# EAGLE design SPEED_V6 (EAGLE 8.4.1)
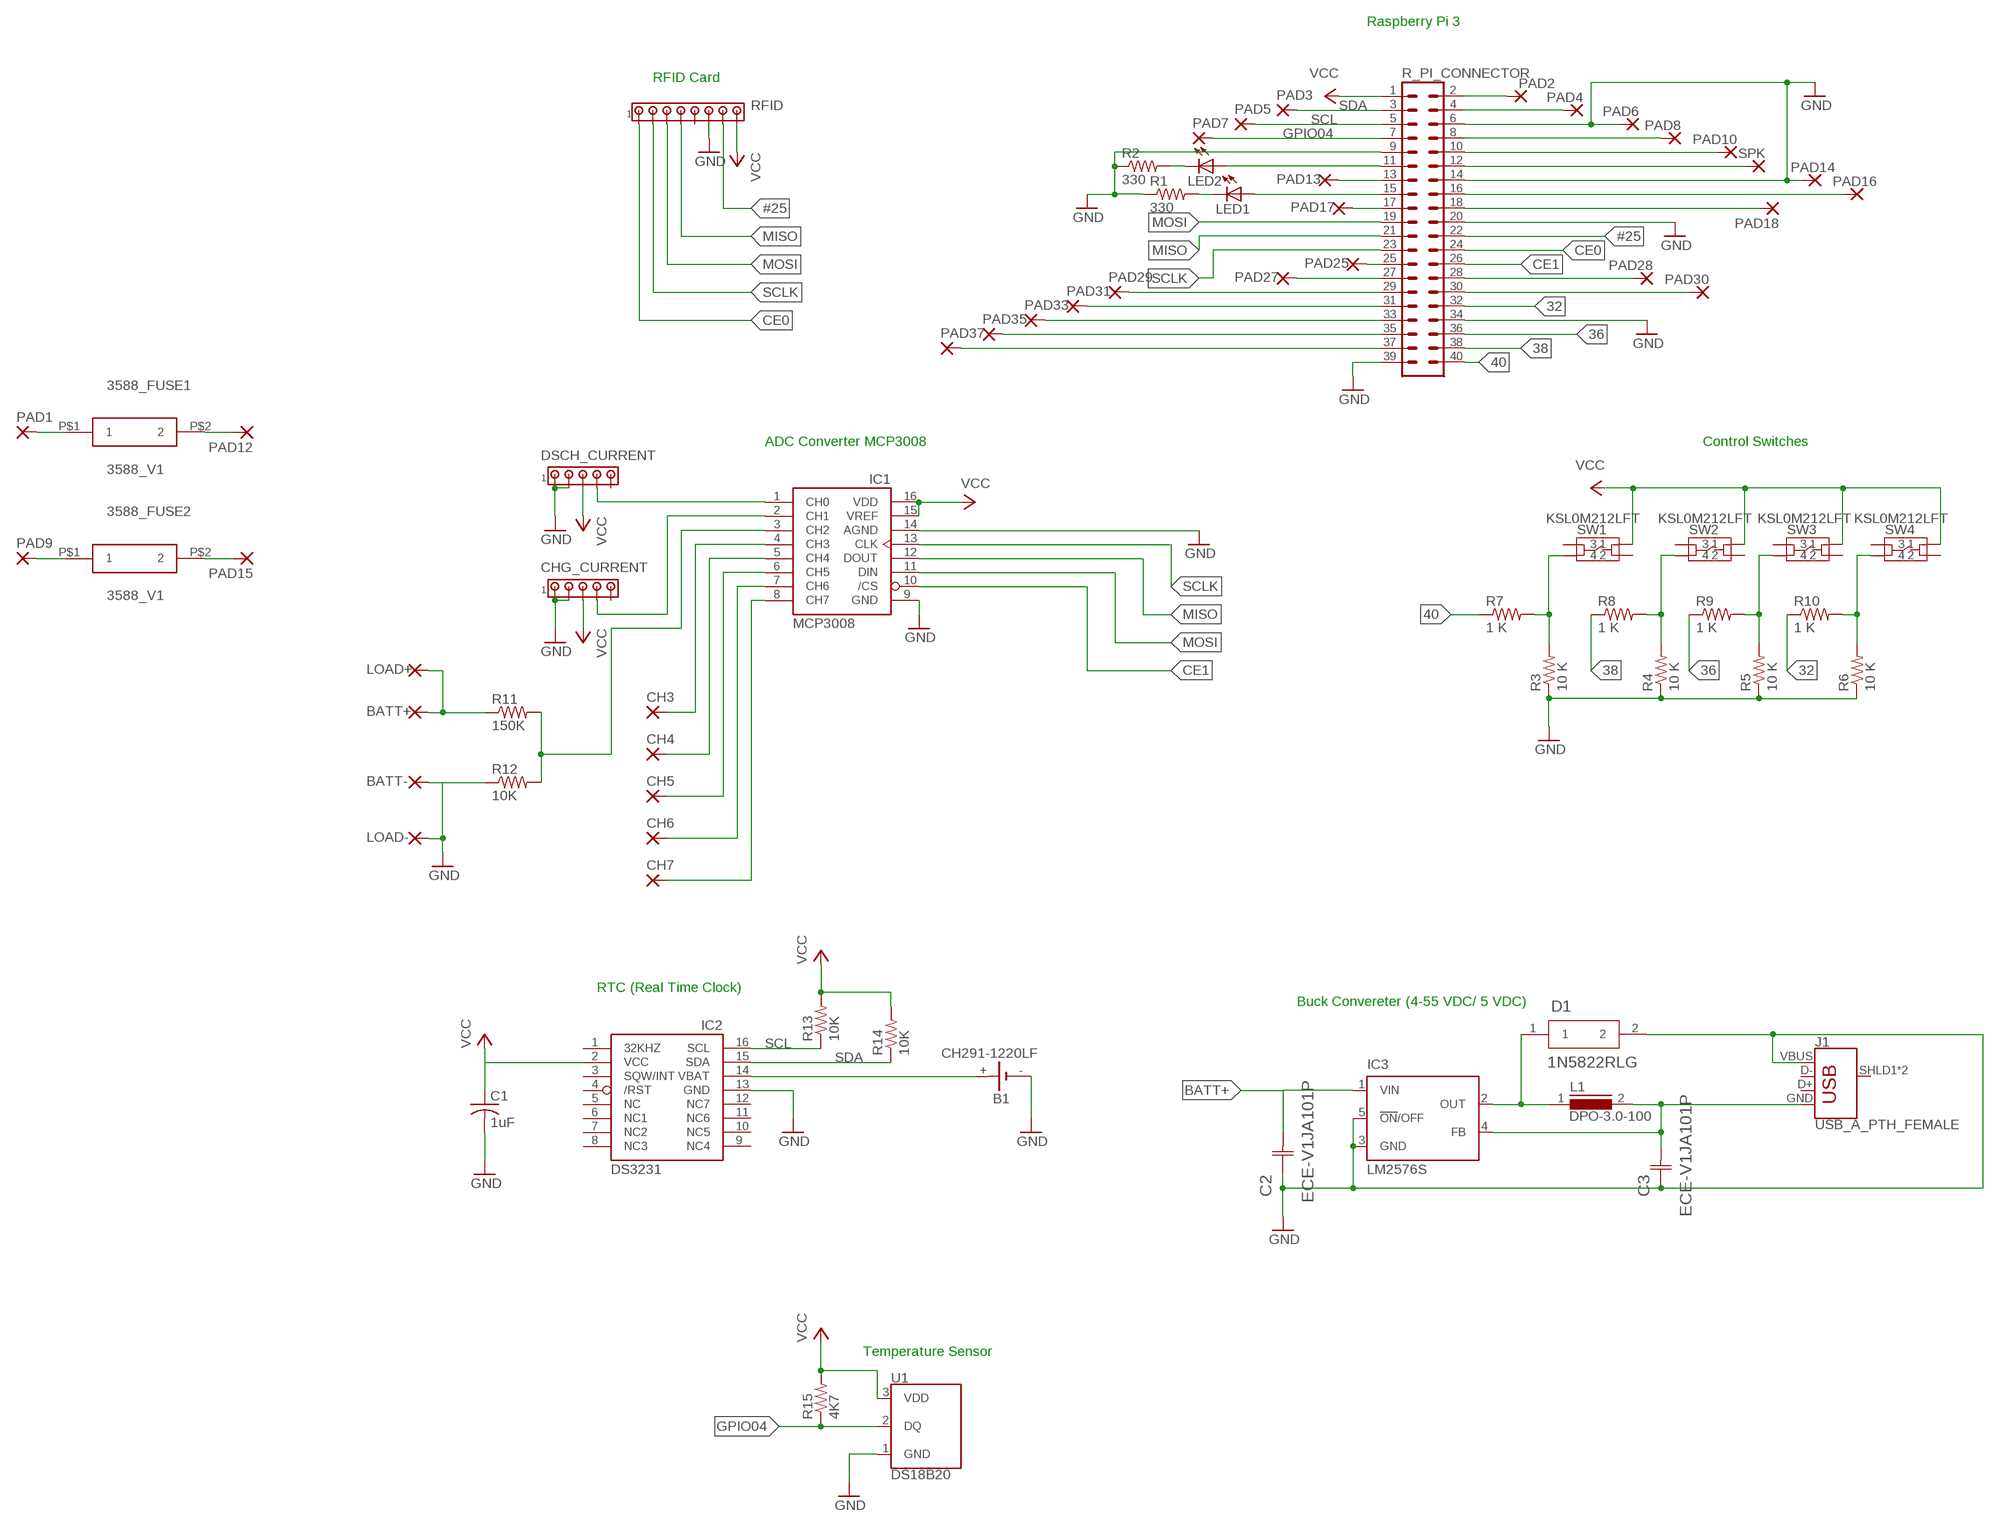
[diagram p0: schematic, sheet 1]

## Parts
3588_FUSE1  3588_V1  [3588_V1]
3588_FUSE2  3588_V1  [3588_V1]
B1  CH291-1220LF  [CH291-1220LF]
BATT+  3,81/1,4  [3,81/1,4]
BATT-  3,81/1,4  [3,81/1,4]
C1  1uF  C-USC0805  [C0805]
C2  ECE-V1JA101P  [CAP_ECEV_G]
C3  ECE-V1JA101P  [CAP_ECEV_G]
CH3  WIREPAD1,6/0,9  [1,6/0,9]
CH4  WIREPAD1,6/0,9  [1,6/0,9]
CH5  WIREPAD1,6/0,9  [1,6/0,9]
CH6  WIREPAD1,6/0,9  [1,6/0,9]
CH7  WIREPAD1,6/0,9  [1,6/0,9]
CHG_CURRENT  MTA05-100  [10X05MTA]
D1  1N5822RLG  [CASE_267-05]
DSCH_CURRENT  MTA05-100  [10X05MTA]
IC1  MCP3008  [DIL16]
IC2  DS3231/SO  [SO16W]
IC3  LM2576S  LM2596S  [TO263-5]
J1  USB_A_PTH_FEMALE  USB_A_PTH_MALE  [USB-A-H]
L1  DPO-3.0-100  ED26  [ED26]
LED1  LED5MM  [LED5MM]
LED2  LED5MM  [LED5MM]
LOAD+  3,81/1,4  [3,81/1,4]
LOAD-  3,81/1,4  [3,81/1,4]
PAD1  3,81/1,4  [3,81/1,4]
PAD2  1,6/0,9  [1,6/0,9]
PAD3  1,6/0,9  [1,6/0,9]
PAD4  1,6/0,9  [1,6/0,9]
PAD5  1,6/0,9  [1,6/0,9]
PAD6  1,6/0,9  [1,6/0,9]
PAD7  1,6/0,9  [1,6/0,9]
PAD8  1,6/0,9  [1,6/0,9]
PAD9  3,81/1,4  [3,81/1,4]
PAD10  1,6/0,9  [1,6/0,9]
PAD12  3,81/1,4  [3,81/1,4]
PAD13  1,6/0,9  [1,6/0,9]
PAD14  WIREPAD1,6/0,9  [1,6/0,9]
PAD15  3,81/1,4  [3,81/1,4]
PAD16  1,6/0,9  [1,6/0,9]
PAD17  1,6/0,9  [1,6/0,9]
PAD18  1,6/0,9  [1,6/0,9]
PAD25  1,6/0,9  [1,6/0,9]
PAD27  1,6/0,9  [1,6/0,9]
PAD28  1,6/0,9  [1,6/0,9]
PAD29  1,6/0,9  [1,6/0,9]
PAD30  1,6/0,9  [1,6/0,9]
PAD31  1,6/0,9  [1,6/0,9]
PAD33  1,6/0,9  [1,6/0,9]
PAD35  1,6/0,9  [1,6/0,9]
PAD37  1,6/0,9  [1,6/0,9]
R1  330  R-US_R1206  [R1206]
R2  330  R-US_R1206  [R1206]
R3  10 K  R-US_R1206  [R1206]
R4  10 K  R-US_R1206  [R1206]
R5  10 K  R-US_R1206  [R1206]
R6  10 K  R-US_R1206  [R1206]
R7  1 K  R-US_R1206  [R1206]
R8  1 K  R-US_R1206  [R1206]
R9  1 K  R-US_R1206  [R1206]
R10  1 K  R-US_R1206  [R1206]
R11  150K  R-US_R1206  [R1206]
R12  10K  R-US_R1206  [R1206]
R13  10K  R-US_R1206  [R1206]
R14  10K  R-US_R1206  [R1206]
R15  4K7  R-US_R1206  [R1206]
R_PI_CONNECTOR  SBH11-PBPC-D20  [SBH11-PBPC-D20]
RFID  MTA08-100  [10X08MTA]
SPK  WIREPAD1,6/0,9  [1,6/0,9]
SW1  KSL0M212LFT  [KSL0M212LFT_SWITCH]
SW2  KSL0M212LFT  [KSL0M212LFT_SWITCH]
SW3  KSL0M212LFT  [KSL0M212LFT_SWITCH]
SW4  KSL0M212LFT  [KSL0M212LFT_SWITCH]
U1  DS18B20  [TO-92-AMMO]

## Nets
32: R10.1 R_PI_CONNECTOR.32
36: R9.1 R_PI_CONNECTOR.36
38: R8.1 R_PI_CONNECTOR.38
40: R7.1 R_PI_CONNECTOR.40
#25: R_PI_CONNECTOR.22 RFID.7
BATT+: BATT+.1(P) C2.2 IC3.1(VIN) LOAD+.1(P) R11.1
CE0: R_PI_CONNECTOR.24 RFID.1
CE1: IC1.10(/CS) R_PI_CONNECTOR.26
GND: B1.- BATT-.1(P) C1.2 C2.1 C3.1 CHG_CURRENT.1 CHG_CURRENT.2 D1.2 DSCH_CURRENT.1 DSCH_CURRENT.2 IC1.9(GND) IC1.14(AGND) IC2.13(GND) IC3.3(GND) IC3.5(!ON!/OFF) J1.VBUS LOAD-.1(P) PAD6.1(P) PAD14.1(P) R1.1 R2.1 R3.1 R4.1 R5.1 R6.1 R12.1 R_PI_CONNECTOR.6 R_PI_CONNECTOR.9 R_PI_CONNECTOR.14 R_PI_CONNECTOR.20 R_PI_CONNECTOR.34 R_PI_CONNECTOR.39 RFID.6 U1.1(GND)
GPIO04: PAD7.1(P) R15.1 R_PI_CONNECTOR.7 U1.2(DQ)
MISO: IC1.12(DOUT) R_PI_CONNECTOR.21 RFID.4
MOSI: IC1.11(DIN) R_PI_CONNECTOR.19 RFID.3
N$1: R_PI_CONNECTOR.12 SPK.1(P)
N$2: PAD28.1(P) R_PI_CONNECTOR.28
N$3: LED1.K(C) R1.2
N$4: LED1.A R_PI_CONNECTOR.15
N$5: R6.2 R10.2 SW4.P$4
N$6: DSCH_CURRENT.4 IC1.1(CH0)
N$7: CHG_CURRENT.4 IC1.2(CH1)
N$8: IC1.3(CH2) R11.2 R12.2
N$9: PAD30.1(P) R_PI_CONNECTOR.30
N$10: PAD18.1(P) R_PI_CONNECTOR.18
N$11: PAD10.1(P) R_PI_CONNECTOR.10
N$12: PAD8.1(P) R_PI_CONNECTOR.8
N$13: 3588_FUSE1.P$1 PAD1.1(P)
N$14: D1.1 IC3.2(OUT) L1.1
N$15: PAD4.1(P) R_PI_CONNECTOR.4
N$16: R5.2 R9.2 SW3.P$4
N$17: LED2.A R_PI_CONNECTOR.11
N$18: LED2.K(C) R2.2
N$19: R4.2 R8.2 SW2.P$4
N$20: R3.2 R7.2 SW1.P$4
N$21: PAD2.1(P) R_PI_CONNECTOR.2
N$22: PAD13.1(P) R_PI_CONNECTOR.13
N$23: PAD17.1(P) R_PI_CONNECTOR.17
N$24: B1.+ IC2.14(VBAT)
N$25: PAD25.1(P) R_PI_CONNECTOR.25
N$26: PAD27.1(P) R_PI_CONNECTOR.27
N$27: PAD29.1(P) R_PI_CONNECTOR.29
N$28: PAD31.1(P) R_PI_CONNECTOR.31
N$29: PAD33.1(P) R_PI_CONNECTOR.33
N$30: PAD35.1(P) R_PI_CONNECTOR.35
N$31: PAD37.1(P) R_PI_CONNECTOR.37
N$32: PAD16.1(P) R_PI_CONNECTOR.16
N$33: 3588_FUSE1.P$2 PAD12.1(P)
N$34: CH3.1(P) IC1.4(CH3)
N$35: CH4.1(P) IC1.5(CH4)
N$36: CH5.1(P) IC1.6(CH5)
N$37: CH6.1(P) IC1.7(CH6)
N$38: CH7.1(P) IC1.8(CH7)
N$39: C3.2 IC3.4(FB) J1.GND L1.2
N$40: 3588_FUSE2.P$1 PAD9.1(P)
N$41: 3588_FUSE2.P$2 PAD15.1(P)
SCL: IC2.16(SCL) PAD5.1(P) R13.1 R_PI_CONNECTOR.5
SCLK: IC1.13(CLK) R_PI_CONNECTOR.23 RFID.2
SDA: IC2.15(SDA) PAD3.1(P) R14.1 R_PI_CONNECTOR.3
VCC: C1.1 CHG_CURRENT.3 DSCH_CURRENT.3 IC1.15(VREF) IC1.16(VDD) IC2.2(VCC) R13.2 R14.2 R15.2 R_PI_CONNECTOR.1 RFID.8 SW1.P$2 SW2.P$2 SW3.P$2 SW4.P$2 U1.3(VDD)
Unconnected: CHG_CURRENT.5 DSCH_CURRENT.5 IC2.1(32KHZ) IC2.3(SQW/INT) IC2.4(/RST) IC2.5(NC) IC2.6(NC1) IC2.7(NC2) IC2.8(NC3) IC2.9(NC4) IC2.10(NC5) IC2.11(NC6) IC2.12(NC7) J1.D+ J1.D- J1.SHLD1(SHIELD) J1.SHLD2(SHIELD) RFID.5 SW1.P$1 SW1.P$3 SW2.P$1 SW2.P$3 SW3.P$1 SW3.P$3 SW4.P$1 SW4.P$3

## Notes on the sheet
- Raspberry Pi 3
- RFID Card
- ADC Converter MCP3008 | Control Switches
- RTC (Real Time Clock)
- Buck Convereter (4-55 VDC/ 5 VDC)
- Temperature Sensor

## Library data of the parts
3588_FUSE1 3588_FUSE2 = costin_1:3588_V1
B1 = battery:CH291-1220LF: Battery Holder, SMT, 12mm
BATT+ = wirepad:3,81/1,4: THROUGH-HOLE PAD; SPICEPREFIX: X
BATT- LOAD+ LOAD- PAD1 PAD9 PAD12 PAD15 = wirepad:3,81/1,4: THROUGH-HOLE PAD
C1 = adafruit:C-US: CAPACITOR, American symbol
C2 C3 = digikey1:ECE-V1JA101P; MANUFACTURER_PART_NUMBER: ECEV1JA101P; VENDOR: Panasonic
CH3-CH7 PAD14 SPK = wirepad:WIREPAD: Wire PAD connect wire on PCB
CHG_CURRENT DSCH_CURRENT = con-amp:MTA05-100: AMP connector
D1 = digikey1:1N5822RLG; MANUFACTURER_PART_NUMBER: 1N5822RLG; VENDOR: ON Semiconductor
IC1 = adafruit:MCP3008
IC2 = adafruit:DS3231
IC3 = national-semiconductor:LM2596: SIMPLE SWITCHER® Power Converter 150 kHz 3A Step-Down Voltage Regulator Source: http://www.national.com/ds/LM/LM2596.pdf; MF: NATIONAL SEMICONDUCTOR; MPN: LM2596S-ADJ/NOPB; OC_FARNELL: 9494367; OC_NEWARK: 41K3842
J1 = SparkFun-Connectors:USB_A: USB-A Connector Male and female variants, as well as PTH and SMT variants SparkFun Products: SparkFun XBee Explorer Dongle PTH Male SparkFun MicroView-USB Programmer SMT Male SparkFun USB Type A Female Breakout SMT Female; PROD_ID: CONN-08367; SF_ID: PRT-00437; SPICEPREFIX: X
L1 = inductors:ED26: INDUCTOR; SPICEPREFIX: L
LED1 LED2 = adafruit:LED: LED
PAD2-PAD8 PAD10 PAD13 PAD16-PAD18 PAD25 PAD27-PAD31 PAD33 PAD35 PAD37 = wirepad:1,6/0,9: THROUGH-HOLE PAD
R1 R2 R11-R15 = adafruit:R-US_: RESISTOR, American symbol
R3-R6 = adafruit:R-US_: RESISTOR, American symbol; MPN: RC1206JR-0710KL; OC_NEWARK: 68R0303
R7-R10 = adafruit:R-US_: RESISTOR, American symbol; OC_NEWARK: unknown
R_PI_CONNECTOR = con-sullins:SBH11-PBPC-D20: HEADER - Vertical, Shrouded
RFID = con-amp:MTA08-100: AMP connector
SW1-SW4 = costin_1:KSL0M212LFT
U1 = SparkFun-Sensors:DS18B20: Dallas/Maxim DS18B20 1-Wire Temperature Sensor The DS18B20 reports degrees C with 9 to 12-bit precision, -55C to 125C (+/-0.5C). Each sensor has a unique 64-Bit Serial number etched into it - allows for a huge number of sensors to be used on one data bus. Datasheet SparkFun Products One Wire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; STORE_ID: SEN-00245

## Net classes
0 default: width 0.305 mm, drill 0.508 mm, clearance 0.254 mm

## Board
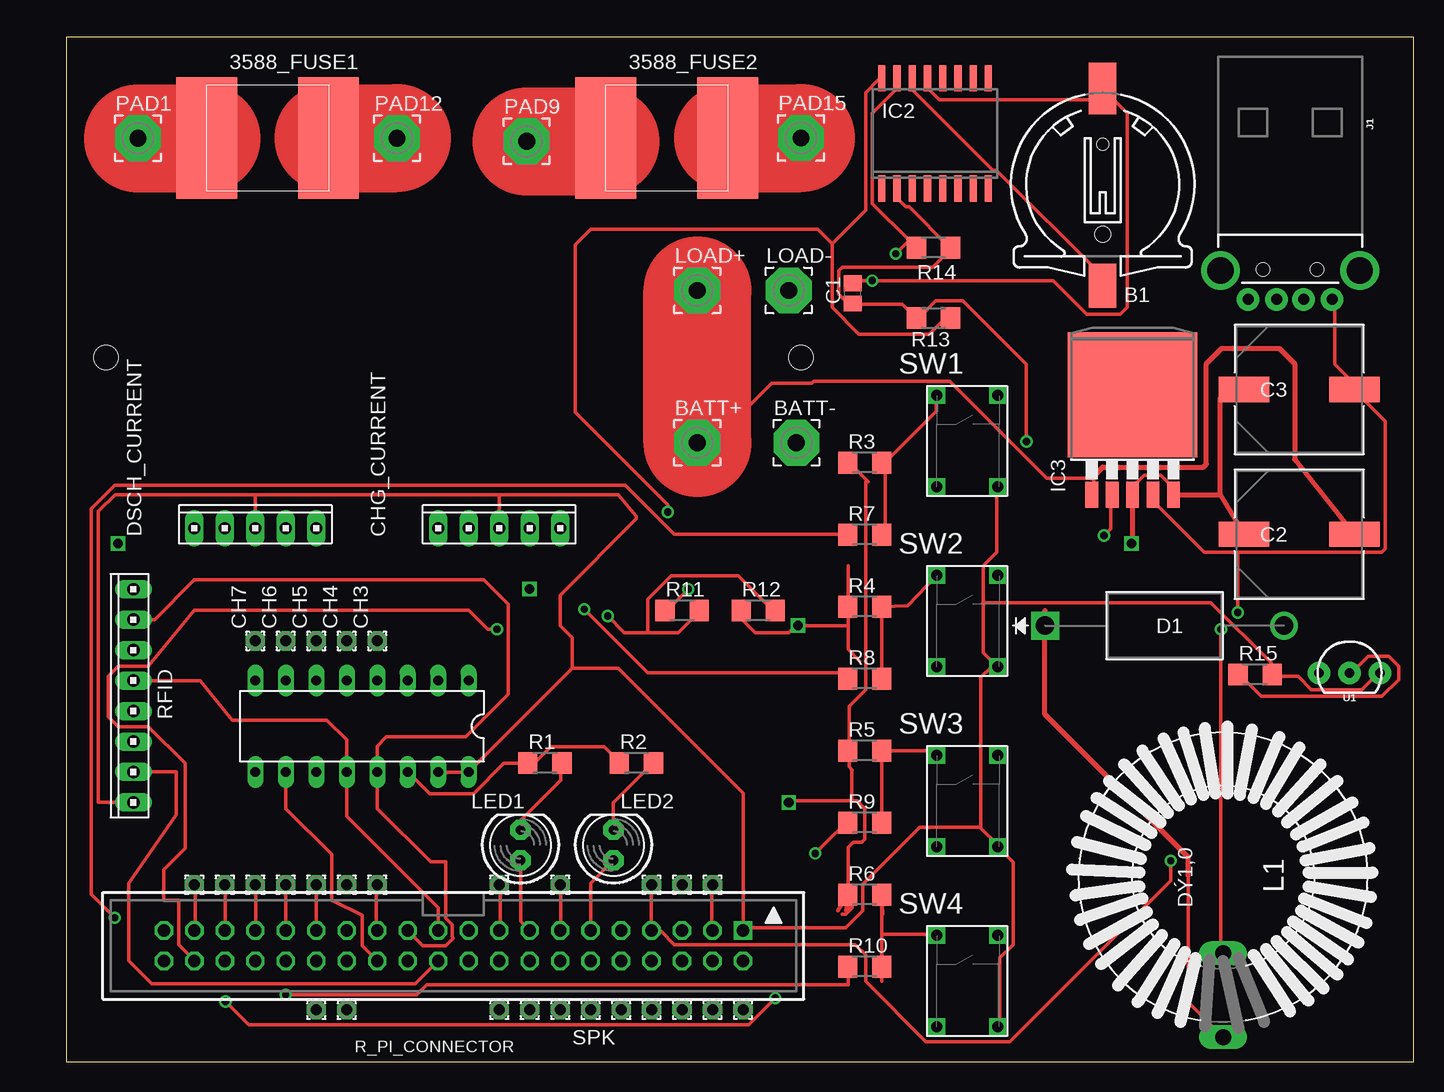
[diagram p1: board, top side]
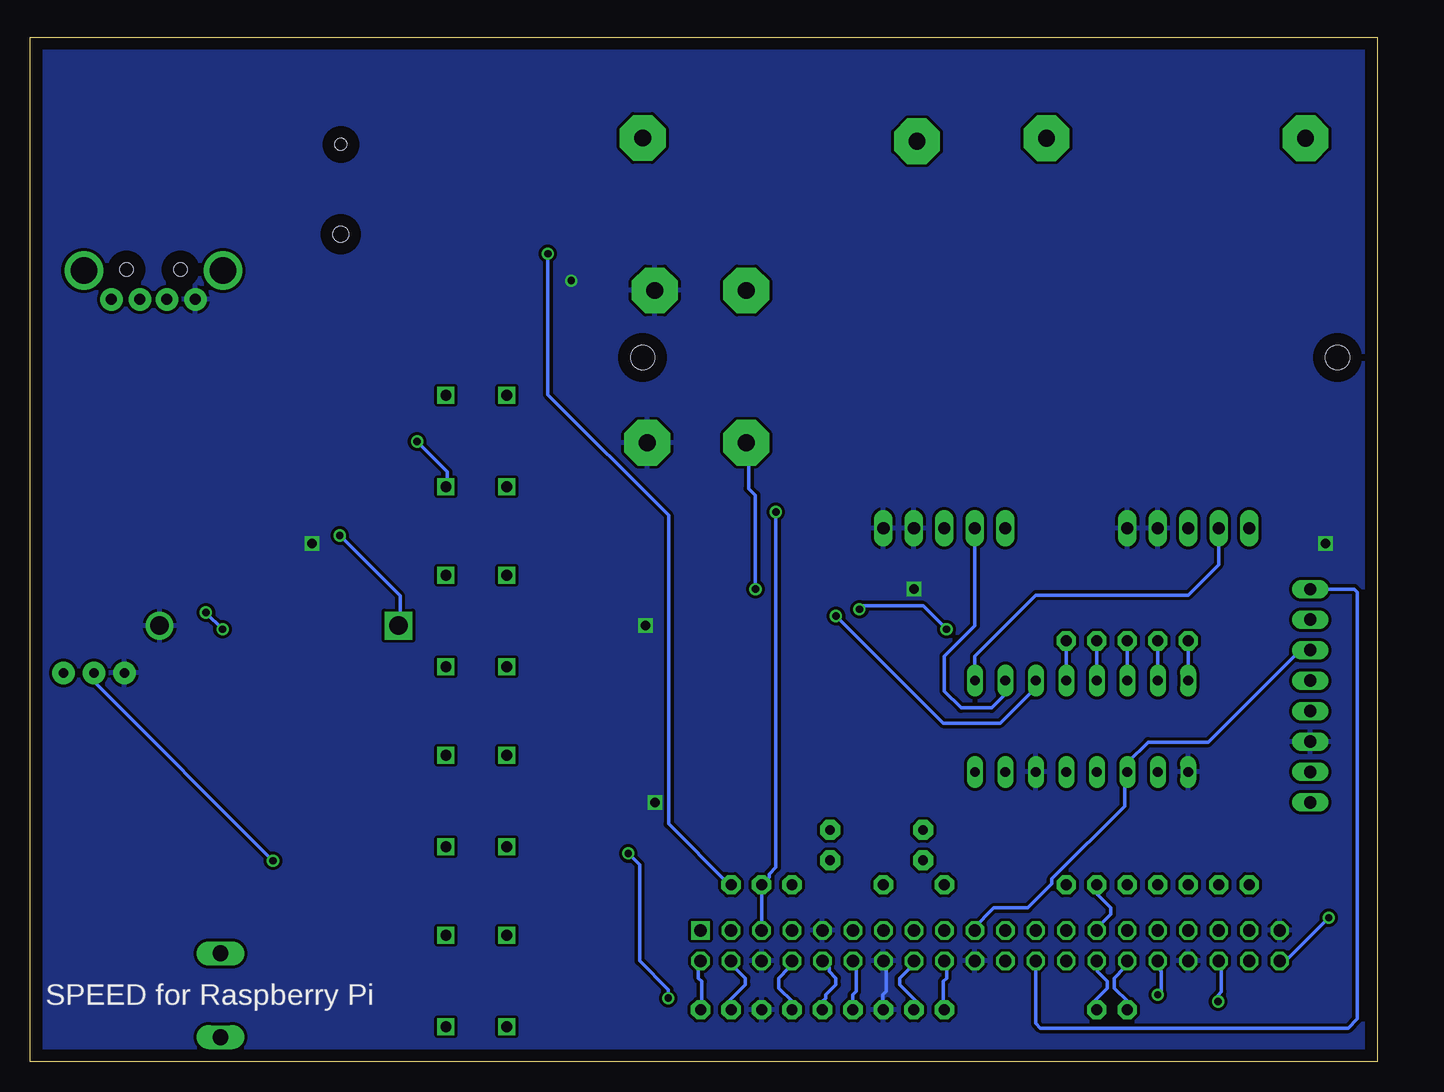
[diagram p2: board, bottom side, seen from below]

Size 112.27 x 85.34 mm. Coordinates in mm from the lower left corner, seen from the top.
Outline: 0,0 112.27,0 112.27,85.34 0,85.34 0,0
Copper layers (1*16): Top 0.035mm / dielectric 1.5mm / Bottom 0.035mm
Design rules "default": minimum track width 10mil, minimum drill 24mil, track to track 8mil, track to pad 8mil, pad to pad 8mil, via to via 8mil, smd to smd 8mil, copper to edge 40mil, drill to drill 8mil, minimum pad ring 10mil, minimum via ring 8mil, stop-mask expansion 4mil, vias tented up to drill 0mil, thermal gap 10mil
Holes 2 mm at 3.3,58.67 61.21,58.67

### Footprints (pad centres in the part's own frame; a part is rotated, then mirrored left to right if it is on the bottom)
3588_V1 = smd 5.08 x 10.16: P$1 -5.08,0; P$2 5.08,0
CH291-1220LF = smd 2.3 x 3.66: + 0,-2.296 | smd 2.3 x 4.3: - 0,14.146 | hole 1.3: 0,2 | hole 1: 0,9.5
3,81/1,4 = drill 1.397 pad 3.81 octagon: 1 0,0
C0805 = smd 1.3 x 1.5: 1 -0.85,0; 2 0.85,0
CAP_ECEV_G = smd 4.216 x 2.108: 1 -4.597,0; 2 4.597,0
1,6/0,9 = drill 0.914 pad 1.6 octagon: 1 0,0
10X05MTA = drill 1.016 long: 1 5.08,0; 2 2.54,0; 3 0,0; 4 -2.54,0; 5 -5.08,0
CASE_267-05 = drill 1.549 pad 2.057 square: 1 -19.914,0 | drill 1.549 pad 2.057: 2 0,0
DIL16 = drill 0.813 long: 1 -8.89,-3.81; 2 -6.35,-3.81; 3 -3.81,-3.81; 4 -1.27,-3.81; 5 1.27,-3.81; 6 3.81,-3.81; 7 6.35,-3.81; 8 8.89,-3.81; 9 8.89,3.81; 10 6.35,3.81; 11 3.81,3.81; 12 1.27,3.81; 13 -1.27,3.81; 14 -3.81,3.81; 15 -6.35,3.81; 16 -8.89,3.81
SO16W = smd 0.6 x 2.2: 1 -4.445,-4.6; 2 -3.175,-4.6; 3 -1.905,-4.6; 4 -0.635,-4.6; 5 0.635,-4.6; 6 1.905,-4.6; 7 3.175,-4.6; 8 4.445,-4.6; 9 4.445,4.6; 10 3.175,4.6; 11 1.905,4.6; 12 0.635,4.6; 13 -0.635,4.6; 14 -1.905,4.6; 15 -3.175,4.6; 16 -4.445,4.6
TO263-5 = smd 1.067 x 2.159: 1 -3.404,-5.791; 2 -1.702,-5.791; 3 0,-5.791; 4 1.702,-5.791; 5 3.404,-5.791 | smd 10.8 x 10.41: 6 0,2.54
USB-A-H = drill 0.914 pad 1.88: D+ 2.4,1.127; D- 2.4,-1.127; GND 2.4,3.5; VBUS 2.4,-3.5 | drill 2.2: SHLD1 0,-5.8; SHLD2 0,5.8 | hole 1.1: -0.1,2.25; -0.1,-2.25
ED26 = drill 1.321 long: 1 -13.335,0; 2 -6.35,0
LED5MM = drill 0.813 pad 1.676 octagon: A -1.27,0; K 1.27,0
R1206 = smd 1.6 x 1.803: 1 -1.422,0; 2 1.422,0
SBH11-PBPC-D20 = drill 1.016 square: 1 -24.13,-1.27 | drill 1.016 octagon: 2 -24.13,1.27; 3 -21.59,-1.27; 4 -21.59,1.27; 5 -19.05,-1.27; 6 -19.05,1.27; 7 -16.51,-1.27; 8 -16.51,1.27; 9 -13.97,-1.27; 10 -13.97,1.27; 11 -11.43,-1.27; 12 -11.43,1.27; 13 -8.89,-1.27; 14 -8.89,1.27; 15 -6.35,-1.27; 16 -6.35,1.27; 17 -3.81,-1.27; 18 -3.81,1.27; 19 -1.27,-1.27; 20 -1.27,1.27; 21 1.27,-1.27; 22 1.27,1.27; 23 3.81,-1.27; 24 3.81,1.27; 25 6.35,-1.27; 26 6.35,1.27; 27 8.89,-1.27; 28 8.89,1.27; 29 11.43,-1.27; 30 11.43,1.27; 31 13.97,-1.27; 32 13.97,1.27; 33 16.51,-1.27; 34 16.51,1.27; 35 19.05,-1.27; 36 19.05,1.27; 37 21.59,-1.27; 38 21.59,1.27; 39 24.13,-1.27; 40 24.13,1.27
10X08MTA = drill 1.016 long: 1 8.89,0; 2 6.35,0; 3 3.81,0; 4 1.27,0; 5 -1.27,0; 6 -3.81,0; 7 -6.35,0; 8 -8.89,0
KSL0M212LFT_SWITCH = drill 0.9 square: P$1 0,0; P$2 5.08,0; P$3 5.08,7.62; P$4 0,7.62
TO-92-AMMO = drill 0.813 pad 1.88: 1 -2.54,0; 2 0,0; 3 2.54,0

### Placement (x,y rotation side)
3588_FUSE1  16.76,76.96 0 top
3588_FUSE2  50.04,76.96 0 top
B1  86.36,66.93 0 top
BATT+  52.58,51.56 0 top
BATT-  60.83,51.56 0 top
C1  65.53,64.01 90 top
C2  102.74,43.94 0 top
C3  102.74,56.01 0 top
CH3  25.91,35.05 0 top
CH4  23.37,35.05 0 top
CH5  20.83,35.05 0 top
CH6  18.29,35.05 0 top
CH7  15.75,35.05 0 top
CHG_CURRENT  36.07,44.45 0 top
D1  101.47,36.32 0 top
DSCH_CURRENT  15.75,44.45 0 top
IC1  24.64,27.94 180 top
IC2  72.39,77.34 0 top
IC3  88.85,53.01 0 top
J1  101.98,65.91 270 top
L1  96.39,15.37 90 top
LED1  37.85,18.03 90 top
LED2  45.59,18.03 90 top
LOAD+  52.58,64.26 0 top
LOAD-  60.2,64.26 0 top
PAD1  5.97,76.94 0 top
PAD2  56.39,4.32 0 top
PAD3  53.85,14.73 0 top
PAD4  53.85,4.32 0 top
PAD5  51.31,14.73 0 top
PAD6  51.31,4.32 0 top
PAD7  48.77,14.73 0 top
PAD8  48.77,4.32 0 top
PAD9  38.35,76.68 0 top
PAD10  46.23,4.32 0 top
PAD12  27.56,76.94 0 top
PAD13  41.15,14.73 0 top
PAD14  41.15,4.32 0 top
PAD15  61.21,76.96 0 top
PAD16  38.61,4.32 0 top
PAD17  36.07,14.73 0 top
PAD18  36.07,4.32 0 top
PAD25  25.91,14.73 0 top
PAD27  23.37,14.73 0 top
PAD28  23.37,4.32 0 top
PAD29  20.83,14.73 0 top
PAD30  20.83,4.32 0 top
PAD31  18.29,14.73 0 top
PAD33  15.75,14.73 0 top
PAD35  13.21,14.73 0 top
PAD37  10.67,14.73 0 top
R1  39.88,24.89 0 top
R2  47.5,24.89 0 top
R3  66.53,49.9 0 top
R4  66.53,37.9 0 top
R5  66.53,25.9 0 top
R6  66.53,13.9 0 top
R7  66.53,43.9 0 top
R8  66.53,31.9 0 top
R9  66.53,19.9 0 top
R10  66.53,7.9 0 top
R11  51.31,37.59 0 top
R12  57.66,37.59 0 top
R13  72.26,61.98 180 top
R14  72.26,67.82 0 top
R15  99.06,32.26 0 top
R_PI_CONNECTOR  32.26,9.65 180 top
RFID  5.59,30.48 90 top
SPK  43.69,4.32 0 top
SW1  72.53,47.9 0 top
SW2  72.53,32.9 0 top
SW3  72.53,17.9 0 top
SW4  72.53,2.9 0 top
U1  106.93,32.38 0 top

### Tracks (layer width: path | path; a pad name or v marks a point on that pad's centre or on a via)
32  (via drill 0.61)
  Top 0.305: v18.29,5.56 29.19,5.56 30.02,6.4 65.15,6.4 R10.1
  Bottom 0.305: R_PI_CONNECTOR.32 18.29,7.8 18.01,7.52 18.01,5.82 18.27,5.55 | 18.29,5.54 18.27,5.55 | v18.29,5.56 18.27,5.55
36  (via drill 0.61)
  Top 0.305: v62.41,17.35 64.03,18.97 R9.1 | v59.08,5.28 56.84,3.05 15.22,3.05 v13.26,5
  Bottom 0.305: 13.26,4.98 v13.26,5 13.26,5.54 12.98,5.82 12.98,8.36 R_PI_CONNECTOR.36 | v59.08,5.28 59.08,5.99 61.47,8.38 61.47,16.41 v62.41,17.35
38  (via drill 0.61)
  Top 0.305: v43.16,37.69 48.46,32.38 64.87,32.38 R8.1 | R_PI_CONNECTOR.38 10.47,8.64 9.35,9.75 9.35,13.46 8.13,13.46 8.13,16 9.91,17.78 9.91,24.84 6.83,27.91 4.32,27.91 3.48,28.75 3.48,32.11 4.32,32.94 6.83,32.94 10.67,37.59 33.53,37.59 35.1,36.02 v35.89,36.02
  Bottom 0.305: v43.16,37.69 42.88,37.97 37.85,37.97 v35.89,36.02
40  (via drill 0.61)
  Top 0.305: v4.04,11.99 2.08,13.95 2.08,46.08 4.04,48.03 46.58,48.03 50.67,43.94 65.23,43.94 | 65.23,43.94 65.25,43.94 | R7.1 65.23,43.84 65.23,43.94
  Bottom 0.305: v4.04,11.99 7.39,8.64 7.95,8.64 R_PI_CONNECTOR.40
#25
  Top 0.305: R_PI_CONNECTOR.22 29.08,6.48 7.11,6.48 5.21,8.38 5.21,14.86 9.14,20.57 9.14,24.13 RFID.7
BATT+  (via drill 0.61)
  Top 0.305: 50.14,37.41 R11.1 50.14,37.69 v51.82,39.37 | IC3.1 85.62,47.47 85.62,48.59 85.52,48.69 | 55.12,50.55 52.65,50.55 BATT+.1 52.35,50.55 | 55.12,50.55 56.01,50.55 | 85.45,48.62 85.34,48.59 81.71,48.59 73.61,56.69 62.3,56.69 62.11,56.51 58.79,56.51 55.12,52.83 55.12,50.55
  Top 0.406: C2.2 102.36,50.19 102.36,58.17 101.09,59.44 96.27,59.44 95,58.17 95,49.78 94.74,49.53 86.36,49.53 85.52,48.69 85.45,48.62
  Top 9: BATT+.1 LOAD+.1
  Bottom 0.305: v51.82,39.37 51.82,47.19 52.38,47.75 52.38,50.27 BATT+.1
CE0
  Bottom 0.305: R_PI_CONNECTOR.24 28.45,3.18 28.07,2.79 2.41,2.79 1.65,3.56 1.65,39.12 1.91,39.37 RFID.1
CE1
  Top 0.305: R_PI_CONNECTOR.26 24.64,9.65 24.64,12.19 22.1,13.46 22.1,17.27 18.29,21.08 IC1.10
GND  (via drill 0.61, 0.8)
  Top 0.305: 65.15,41.33 65.15,37.97 | 65.43,49.71 66.73,48.41 | 66.73,48.41 66.83,48.31 | 65.43,49.71 R3.1 65.28,49.89 | 65.15,36.32 65.15,37.97 | 65.15,36.32 65.15,34.34 66.13,33.36 | 65.15,37.97 R4.1 | 65.43,21.72 65.43,24.28 65.51,24.28 65.23,24.56 65.23,25.68 R5.1 65.23,25.96 65.23,29.59 66.62,30.99 66.62,48.31 66.73,48.41 | R6.1 65.15,12.83 65.15,17.86 65.58,18.29 66.29,18.29 66.55,18.54 66.55,21.08 65.91,21.72 65.43,21.72 | 65.15,36.32 v60.96,36.32 60.76,36.3 60.2,35.74 57.4,35.74 56.29,36.86 56.29,37.41 56.26,37.41 R12.1 | R2.1 45.95,25.12 44.83,26.24 40.36,26.24 39.24,25.12 38.68,25.12 R1.1 38.41,24.84 36.45,24.84 33.93,22.33 30.3,22.33 28.63,24 IC1.14 | 64.67,12.27 64.95,12.27 65.23,12.55 | 65.23,12.55 65.51,12.83 R6.1 | R6.1 64.26,12.57 | 65.43,50.44 65.43,49.71 | 65.38,49.66 65.43,49.71 | 65.23,12.55 64.95,12.55 R6.1 | v60.2,21.59 60.32,21.72 65.43,21.72 | IC3.3 88.98,47.47 88.98,48.03 89.81,48.87 91.21,48.87 92.05,48.03 92.05,47.47 IC3.5 | C1.2 65.76,65.08 v67.16,65.08 82.25,65.08 85.04,62.28 87.83,62.28 88.39,62.84 88.39,79.05 86.44,81 B1.- 86.16,81 85.32,80.16 72.75,80.16 71.91,81 71.91,81.84 IC2.13
  Top 0.406: v88.77,43.18 88.85,43.26 IC3.3 | IC3.5 96.14,47.22 | 96.14,47.22 C2.1 | 96.14,47.22 96.14,55.27 C3.1
  Bottom 0.305: R_PI_CONNECTOR.14 40.92,8.36 40.92,5.84 41.2,5.56 41.2,5 PAD14.1
  other vias: 4.32,43.18 38.61,39.37
  pour Bottom: -0.89,86.74 113.41,87 113.41,-0.76 -1.52,-1.02
GPIO04  (via drill 0.61)
  Top 0.305: PAD7.1 48.74,14.5 48.74,11.15 R_PI_CONNECTOR.7 49,10.87 49.55,10.87 50.67,9.75 65.76,9.75 66.6,8.92 66.6,6.68 71.63,1.65 78.61,1.65 92.02,15.06 v92.02,16.74 | R15.1 97.89,32.11 99.57,30.43 109.63,30.43 111.02,31.83 111.02,32.94 110.19,33.78 108.51,33.78 107.11,32.38 U1.2
  Bottom 0.305: v92.02,16.74 106.83,31.55 106.83,32.38 U1.2
MISO
  Top 0.305: RFID.4 11.18,31.75 13.84,28.45 21.72,28.45 23.37,26.8 IC1.12 23.37,20.45 30.99,12.83 R_PI_CONNECTOR.21
MOSI
  Bottom 0.305: R_PI_CONNECTOR.19 33.63,11.12 31.95,12.8 29.11,12.8 27.11,14.8 27.11,15.23 21.06,21.29 21.06,24.11 IC1.11 20.78,24.38 20.78,24.94 19.1,26.62 14.07,26.62 6.53,34.16 5.69,34.16 RFID.3
N$1
  Bottom 0.305: R_PI_CONNECTOR.12 43.43,8.36 43.43,5.84 43.71,5.56 43.71,5 SPK.1
N$2
  Bottom 0.305: R_PI_CONNECTOR.28 23.32,8.36 23.32,7.52 22.48,6.68 22.48,6.12 23.6,5 23.6,4.45 PAD28.1
N$3
  Top 0.305: 37.85,20.07 LED1.K 37.85,20.09 41.2,23.44 41.2,24.84 R1.2
N$4
  Top 0.305: R_PI_CONNECTOR.15 37.85,11.68 LED1.A
N$5
  Top 0.305: 67.94,10.59 67.94,12.55 R6.2 68.02,12.27 | 67.94,10.59 67.94,6.68 R10.2 | 67.94,10.59 72.49,10.59 SW4.P$4
N$6
  Bottom 0.305: DSCH_CURRENT.4 13.21,41.4 15.75,38.86 28.45,38.86 33.53,33.78 IC1.1
N$7
  Bottom 0.305: IC1.2 30.99,30.61 32.13,29.46 34.67,29.46 36.07,30.86 36.07,33.78 33.53,36.32 CHG_CURRENT.4
N$8  (via drill 0.61)
  Top 0.305: 48.46,35.74 46.51,35.74 v45.11,37.13 | 48.46,35.74 50.98,35.74 52.65,37.41 R11.2 | 48.46,35.74 48.46,38.53 50.42,40.49 56.01,40.49 58.8,37.69 R12.2
  Bottom 0.305: v45.11,37.13 36.17,28.19 31.42,28.19 28.63,30.99 28.63,31.55 IC1.3
N$9
  Bottom 0.305: R_PI_CONNECTOR.30 21.08,8.36 21.08,7.8 21.92,6.96 21.92,6.12 20.8,5 20.8,4.45 PAD30.1
N$10
  Bottom 0.305: R_PI_CONNECTOR.18 35.89,8.36 35.89,6.96 36.17,6.68 36.17,4.45 PAD18.1
N$11
  Bottom 0.305: PAD10.1 46.23,5 45.95,5.28 45.95,5.56 45.11,6.4 45.11,6.96 45.67,7.52 45.67,7.8 46.23,8.36 R_PI_CONNECTOR.10
N$12
  Bottom 0.305: R_PI_CONNECTOR.8 49.02,8.36 49.02,7.8 49.86,6.96 49.86,6.12 48.74,5 48.74,4.45 PAD8.1
N$13
  Top 2.54: 11.66,76.94 3588_FUSE1.P$1
  Top 9: PAD1.1 11.66,76.94
N$14  (via drill 0.61)
  Top 0.305: v86.46,43.84 87.02,44.4 87.02,47.19 IC3.2 | L1.1 93.47,4.95 93.47,15.49
  Top 0.406: 93.47,15.49 93.47,17.02 81.53,28.96 81.53,37.57 D1.1
  Bottom 0.305: v86.46,43.84 81.43,38.81 81.43,37.72 D1.1
N$15
  Bottom 0.305: R_PI_CONNECTOR.4 53.77,8.36 53.77,8.08 52.65,6.96 52.65,6.4 54.05,5 54.05,4.45 PAD4.1
N$16
  Top 0.305: R9.2 R5.2 72.15,25.9 SW3.P$4
N$17
  Top 0.305: R_PI_CONNECTOR.11 43.69,14.86 LED2.A
N$18
  Top 0.305: LED2.K 45.59,21.56 R2.2
N$19
  Top 0.305: 67.94,37.69 67.94,37.97 R4.2 | 67.94,37.69 67.94,32.38 R8.2 | 67.94,37.69 R4.2 | R4.2 70.1,37.97 SW2.P$4
N$20
  Top 0.305: R7.2 68.22,44.12 68.22,49.71 R3.2 | 68.5,50.27 68.22,49.99 R3.2 | SW1.P$4 72.49,55.3 72.49,54.18 68.58,50.27 R3.2
N$21
  Bottom 0.305: R_PI_CONNECTOR.2 56.57,8.36 56.57,6.96 56.29,6.68 56.29,4.45 PAD2.1
N$22
  Top 0.305: R_PI_CONNECTOR.13 41.2,11.15 41.2,14.5 PAD13.1
N$23
  Top 0.305: R_PI_CONNECTOR.17 36.17,11.15 36.17,14.5 PAD17.1
N$24
  Top 0.305: IC2.14 70.51,81.84 70.51,81 77.22,74.3 77.5,74.3 86.16,65.63 86.16,64.8 B1.+
N$25
  Top 0.305: R_PI_CONNECTOR.25 25.83,11.15 25.83,14.5 PAD25.1
N$26
  Bottom 0.305: R_PI_CONNECTOR.27 23.32,11.15 22.2,12.27 22.2,12.83 23.32,13.95 23.32,14.5 PAD27.1
N$27
  Top 0.305: R_PI_CONNECTOR.29 20.8,11.15 20.8,14.5 PAD29.1
N$28
  Top 0.305: PAD31.1 R_PI_CONNECTOR.31
N$29
  Top 0.305: R_PI_CONNECTOR.33 15.77,11.15 15.77,14.5 PAD33.1
N$30
  Top 0.305: R_PI_CONNECTOR.35 13.26,11.15 13.26,14.5 PAD35.1
N$31
  Top 0.305: R_PI_CONNECTOR.37 10.74,11.15 10.74,14.5 PAD37.1
N$32
  Bottom 0.305: R_PI_CONNECTOR.16 38.68,8.36 38.68,8.08 39.8,6.96 39.8,6.4 38.41,5 38.41,4.45 PAD16.1
N$33
  Top 2.54: 27.53,76.96 PAD12.1
  Top 9: 3588_FUSE1.P$2 27.53,76.96
N$34
  Bottom 0.305: IC1.4 CH3.1
N$35
  Bottom 0.305: IC1.5 CH4.1
N$36
  Bottom 0.305: IC1.6 CH5.1
N$37
  Bottom 0.305: CH6.1 IC1.7
N$38
  Bottom 0.305: IC1.8 CH7.1
N$39  (via drill 0.61)
  Top 0.305: 96.52,8.92 L1.2 96.22,9.2 v96.22,36.02 | C3.2 107.42,56.41 | 97.61,42.44 109.63,42.44 109.91,42.72 109.91,53.34 107.39,55.86 C3.2 | 97.61,42.44 94.82,42.44 90.63,46.63 90.63,47.19 IC3.4 | J1.GND 105.72,63.4 105.72,58.09 107.39,56.41 C3.2 | 97.61,42.44 v97.61,37.41
  Bottom 0.305: v97.61,37.41 v96.22,36.02
N$40
  Top 2.54: 44.93,76.68 3588_FUSE2.P$1
  Top 9: PAD9.1 44.93,76.68
N$41
  Top 9: 3588_FUSE2.P$2 PAD15.1
SCL  (via drill 0.61)
  Top 0.305: 63.81,68.15 63.81,62.84 66.04,60.6 71.91,60.6 73.03,61.72 73.58,61.72 R13.1 | 63.81,68.15 66.6,70.94 66.6,80.72 67.72,81.84 IC2.16 | v50.11,45.8 50.11,46.41 42.42,54.1 42.42,68.07 43.69,69.34 62.61,69.34 63.81,68.15
  Bottom 0.305: R_PI_CONNECTOR.5 PAD5.1 51.23,14.78 50.67,15.34 50.67,15.62 50.11,16.18 v50.11,45.8
SCLK
  Top 0.305: 5.72,36.96 RFID.2 7.37,36.83 10.67,40.13 34.8,40.13 36.83,38.1 36.83,30.61 33.27,27.05 26.67,27.05 25.91,26.29 IC1.13 25.91,21.08 30.35,16.64 31.62,16.64 31.62,11.94 32.16,11.41 32.16,10.39 32.26,10.29 31.62,9.65 29.72,9.65 R_PI_CONNECTOR.23
SDA  (via drill 0.61)
  Top 0.305: R_PI_CONNECTOR.3 53.77,11.15 53.77,14.5 PAD3.1 | 70.23,68.43 67.16,71.5 67.16,79.05 69.11,81 69.11,81.84 IC2.15 | 70.23,68.43 70.79,67.87 R14.1 70.23,68.43 | 70.23,68.43 v69.11,67.31
  Bottom 0.305: v69.11,67.31 69.11,55.58 59.05,45.52 59.05,19.81 54.03,14.78 PAD3.1
VCC  (via drill 0.61)
  Top 0.305: 30.84,24.38 IC1.15 31.11,24.11 33.35,24.11 IC1.16 42.16,32.77 | RFID.8 2.67,21.59 2.67,45.85 4.06,47.24 15.75,47.24 | 15.75,47.24 36.07,47.24 | 56.26,10.85 56.29,10.87 R_PI_CONNECTOR.1 | 36.07,47.24 45.97,47.24 47.5,45.42 47.5,45.22 41.15,38.86 41.15,36.32 42.16,35.31 42.16,32.77 | DSCH_CURRENT.3 15.75,47.24 | CHG_CURRENT.3 36.07,47.24 | 42.16,32.77 45.97,32.77 56.39,22.35 R_PI_CONNECTOR.1 | 76.4,38.25 76.4,41.33 77.52,42.44 77.52,47.75 SW1.P$2 | 76.4,38.25 76.4,34.06 77.52,32.94 SW2.P$2 77.1,32.9 76.2,32 76.2,19.53 | SW4.P$2 77.8,3.05 77.8,8.64 78.92,9.75 78.92,16.59 SW3.P$2 77.61,18.05 76.2,19.46 76.2,19.53 | 76.2,19.53 71.09,19.53 66.34,14.78 66.34,12.55 64.95,11.15 56.57,11.15 R_PI_CONNECTOR.1 | IC2.2 69.39,72.62 69.39,71.78 69.95,71.22 70.23,71.22 73.58,67.87 R14.2 73.58,67.59 72.19,66.19 64.64,66.19 64.36,65.91 64.36,63.96 64.92,63.4 65.48,63.4 C1.1 65.76,63.12 69.67,63.12 70.79,62 R13.2 71.07,62 72.47,63.4 74.7,63.4 80.01,58.09 v80.01,51.66 | U1.3 109.35,32.38 107.95,30.99 103.76,30.99 102.64,32.11 100.69,32.11 R15.2 100.41,32.38 100.41,33.22 95.38,38.25 76.4,38.25 | 76.38,38.25 76.4,38.25
  Bottom 0.305: v80.01,51.66 77.5,49.15 77.5,48.03 SW1.P$2

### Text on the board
bPlace: SPEED for Raspberry Pi

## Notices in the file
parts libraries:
con-sullins: Copyright (C) 2009, Bob Starr
SparkFun-Connectors: Licensing: Creative Commons ShareAlike 4.0 International - https://creativecommons.org/licenses/by-sa/4.0
